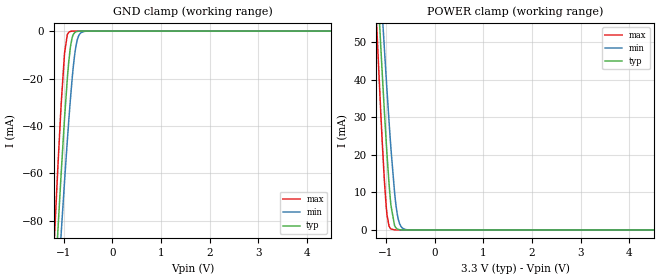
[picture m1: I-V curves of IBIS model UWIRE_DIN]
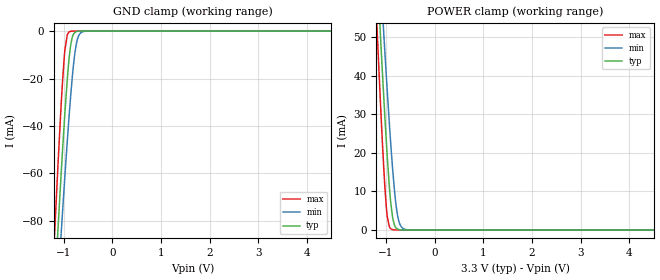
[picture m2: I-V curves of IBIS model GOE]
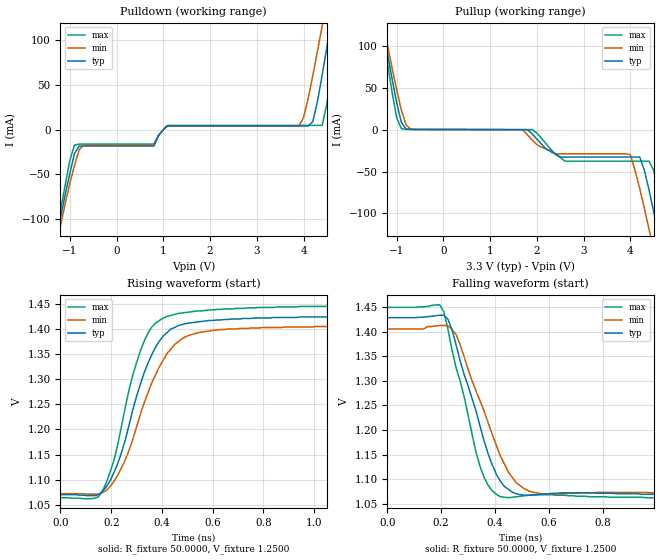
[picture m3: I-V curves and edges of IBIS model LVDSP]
| Texas Instruments Incorporated
| Precision Clock Conditioner with Integrated VCO
| Marketing part#   Voltage Range   Package-type   #pins/pkg drawing
| LMK03001   3.15V - 3.45V   LLP   48-pin SQ
[IBIS Ver]   4.1
[File name]   lmk03001.ibs
[File Rev]   1.4
[Date]   01/28/2014
[Source]   Model built from spectre simulations at:
   Texas Instruments Incorporated.
   Analog-eLab, HPA
   12500 TI Blvd
   Dallas, TX -75243
   For Support e-mail: elab_ibis@list.ti.com
[Notes]   Revision History
   Rev 1.2: 01/28/2014
   - Add uWIRE and GOE buffers, update pin assignments
   Rev 1.0: 3/26/2008
   PullUp and Pulldown non-monotonic for LVPECL and REFOUT models
   LVPECL simulation recommendation:
   It is recommended that a small (1nF or less) AC coupling cap
   be used. Larger values will result in long settling times
[Disclaimer]  This model is designed as an aid for customers of Texas Instruments
 TI and its licensors and suppliers make no warranties, either expressed
 or implied, with respect to this  model, including the warranties of
 merchantability or fitness for a particular purpose.
 The model is provided solely on an "as is" basis. The entire risk as to
 its quality and performance is with the customer.
[Copyright] (C)Copyright 2014 Texas Instruments Incorporated.
[Component]  LMK03001
[Manufacturer]  National Semiconductor Corp
[Package]
|   typ   min   max
R_pkg   0.645   0.430   0.859
L_pkg   1.735nH   1.110nH   2.360nH
C_pkg   0.0455pF   0.037pF   0.054pF
[Pin]   signal_name   model_name   R_pin   L_pin   C_pin
1   GND   GND   0.643   1.770nH   0.054pF
2   Fout   NC   0.531   1.430nH   0.041pF
3   VCC1   POWER   0.482   1.270nH   0.039pF
4   CLKuWire   UWIRE_DIN   0.445   1.160nH   0.039pF
5   DATAuWire   UWIRE_DIN   0.430   1.110nH   0.039pF
6   LEuWire   UWIRE_DIN   0.448   1.160nH   0.039pF
7   NC   NC   0.525   1.390nH   0.043pF
8   VCC2   POWER   0.520   1.370nH   0.039pF
9   LDObyp1   POWER   0.459   1.110nH   0.041pF
10   LDObyp2   POWER   0.462   1.190nH   0.039pF
11   GOE   GOE   0.464   1.220nH   0.041pF
12   LD   NC   0.512   1.390nH   0.053pF
13   VCC3   NC   0.523   1.430nH   0.051pF
14   CLKout0   LVDSP   0.507   1.360nH   0.039pF
15   CLKout0*   LVDSN   0.462   1.220nH   0.037pF
16   VCC4   POWER   0.448   1.170nH   0.037pF
17   CLKout1   LVDSP   0.434   1.120nH   0.037pF
18   CLKout1*   LVDSN   0.443   1.150nH   0.037pF
19   VCC5   POWER   0.470   1.230nH   0.037pF
20   CLKout2   LVDSP   0.505   1.330nH   0.038pF
21   CLKout2*   LVDSN   0.585   1.560nH   0.037pF
22   VCC6   POWER   0.643   1.750nH   0.038pF
23   CLKout3   LVPECLP   0.688   1.900nH   0.039pF
24   CLKout3*   LVPECLN   0.767   2.150nH   0.051pF
25   GND   GND   0.859   2.360nH   0.055pF
26   VCC7   POWER   0.802   2.150nH   0.041pF
27   SYNC*   NC   0.755   2.010nH   0.040pF
28   OSCin   OSCINP   0.725   1.930nH   0.040pF
29   OSCin*   OSCINN   0.711   1.890nH   0.040pF
30   VCC8   POWER   0.710   1.880nH   0.039pF
31   VCC9   POWER   0.745   1.900nH   0.041pF
32   Cpout   NC   0.722   1.920nH   0.040pF
33   VCC10   POWER   0.739   1.960nH   0.040pF
34   NC   NC   0.767   2.050nH   0.040pF
35   NC   NC   0.806   2.170nH   0.041pF
36   BIAS   POWER   0.847   2.330nH   0.054pF
37   VCC11   POWER   0.839   2.340nH   0.051pF
38   CLKout4   LVPECLP   0.821   2.250nH   0.040pF
39   CLKout4*   LVPECLN   0.752   2.030nH   0.038pF
40   VCC12   POWER   0.707   1.900nH   0.038pF
41   CLKout5   LVPECLP   0.670   1.780nH   0.039pF
42   CLKout5*   LVPECLN   0.623   1.650nH   0.038pF
43   VCC13   POWER   0.608   1.610nH   0.039pF
44   CLKout6   LVPECLP   0.606   1.600nH   0.039pF
45   CLKout6*   LVPECLN   0.627   1.660nH   0.038pF
46   VCC14   POWER   0.659   1.760nH   0.039pF
47   CLKout7   LVPECLP   0.695   1.880nH   0.040pF
48   CLKout7*   LVPECLN   0.753   2.080nH   0.051pF
49   DAP   NC
[Diff pin]  inv_pin  vdiff  tdelay_typ  tdelay_min  tdelay_max
14 15   0.0V   0.0s   0.0s   0.0s
17 18   0.0V   0.0s   0.0s   0.0s
20 21   0.0V   0.0s   0.0s   0.0s
23 24   0.0V   0.0s   0.0s   0.0s
28 29   200mV   0.0s   0.0s   0.0s
38 39   0.0V   0.0s   0.0s   0.0s
41 42   0.0V   0.0s   0.0s   0.0s
44 45   0.0V   0.0s   0.0s   0.0s
47 48   0.0V   0.0s   0.0s   0.0s
[Package Model] 48 LLP for LMK03001ISQ AC model at 5 GHz
[Define Package Model]  48 LLP for LMK03001ISQ AC model at 5 GHz
[Manufacturer]   National Semiconductor Corporation
[OEM]   NA
[Description]   48 LLP for LMK03001ISQ, full model
[Number Of Pins]   49
[Pin Numbers]
   1   |   1 = 1
   2   |   2 = 2
   3   |   3 = 3
   4   |   4 = 4
   5   |   5 = 5
   6   |   6 = 6
   7   |   7 = 7
   8   |   8 = 8
   9   |   9 = 9
  10   |  10 = 10
  11   |  11 = 11
  12   |  12 = 12
  13   |  13 = 13
  14   |  14 = 14
  15   |  15 = 15
  16   |  16 = 16
  17   |  17 = 17
  18   |  18 = 18
  19   |  19 = 19
  20   |  20 = 20
  21   |  21 = 21
  22   |  22 = 22
  23   |  23 = 23
  24   |  24 = 24
  25   |  25 = 25
  26   |  26 = 26
  27   |  27 = 27
  28   |  28 = 28
  29   |  29 = 29
  30   |  30 = 30
  31   |  31 = 31
  32   |  32 = 32
  33   |  33 = 33
  34   |  34 = 34
  35   |  35 = 35
  36   |  36 = 36
  37   |  37 = 37
  38   |  38 = 38
  39   |  39 = 39
  40   |  40 = 40
  41   |  41 = 41
  42   |  42 = 42
  43   |  43 = 43
  44   |  44 = 44
  45   |  45 = 45
  46   |  46 = 46
  47   |  47 = 47
  48   |  48 = 48
  49   |  49 = DAP
[Model Data]
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[End Model Data]
[End Package Model]
| Models and submodels in the file (8): UWIRE_DIN (Input), GOE (Input), LVDSP (Output), LVDSN (Output), LVPECLP (Output), LVPECLN (Output), OSCINP (Input), OSCINN (Input)
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|   Model   UWIRE_DIN
[Model] UWIRE_DIN
Model_type Input
Vinh = 0.4V
Vinl = 1.6V
C_comp   0.1674p   0.1674pF   0.1674pF
[Voltage Range]   3.3   3.15   3.45
[Temperature Range]   45   125   -40
[Power Clamp Reference]   3.3   3.15   3.45
[GND Clamp Reference]   0   0   0
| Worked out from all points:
|   GND clamp passes 1 mA (typ) near -0.79 V on its own axis
|   POWER clamp passes 1 mA (typ) near -0.82 V on its own axis
[GND Clamp]
|   Voltage   I(typ)   I(min)   I(max)
-3.3V     -965.6mA   -893.6mA   -1.069A
-1.191V   -112.1mA   -132.7mA   -88.59mA
-1.117V   -84.4mA    -107.7mA   -57.4mA
-1.048V   -59.55mA   -84.92mA   -30.5mA
-978.5mV  -36.37mA   -62.95mA   -9.221mA
-924mV    -20.4mA    -46.56mA   -1.598mA
-859.7mV  -6.75mA    -28.81mA   -125.9uA
-795.3mV  -1.278mA   -14.16mA   -6.168uA
-735.9mV  -231.4uA   -5.307mA   -322.1nA
-681.5mV  -39.54uA   -1.674mA   -19.32nA
-577.5mV  -943.2nA   -148.2uA   0A
6.595V    0A         0A         0A
[POWER Clamp]
|   Voltage   I(typ)   I(min)   I(max)
-3.3V     638.8mA    590.5mA    708.3mA
-1.196V   70.39mA    83.75mA    55.37mA
-1.107V   48.47mA    63.9mA     30.8mA
-1.077V   41.42mA    57.43mA    23.19mA
-1.038V   32.31mA    48.95mA    13.93mA
-978.5mV  19.65mA    36.67mA    3.829mA
-899.2mV  6.493mA    21.57mA    264.8uA
-825mV    1.174mA    9.968mA    10.77uA
-765.6mV  254.2uA    3.922mA    572.9nA
-701.3mV  35.15uA    1.11mA     20.98nA
-582.5mV  494.5nA    81.77uA    0A
6.595V    0A         0A         0A
|   Model GOE
[Model]   GOE
Model_type   Input
Vinl = 0.4
Vinh = 1.6
|   typ   min   max
C_comp   0.3093pF   0.3093pF   0.3093pF
[Voltage Range]   3.3   3.125   3.465
[Temperature Range]   45   125   -40
[Power Clamp Reference]   3.3   3.125   3.465
[GND Clamp Reference]   0   0   0
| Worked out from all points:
|   GND clamp passes 1 mA (typ) near -0.79 V on its own axis
|   POWER clamp passes 1 mA (typ) near -0.82 V on its own axis
[GND Clamp]
|   Voltage   I(typ)   I(min)   I(max)
-3.3V     -965.6mA   -893.6mA   -1.069A
-1.181V   -108.3mA   -129.3mA   -84.35mA
-1.112V   -82.59mA   -106mA     -55.39mA
-1.043V   -57.82mA   -83.32mA   -28.72mA
-973.5mV  -34.81mA   -61.42mA   -8.124mA
-924mV    -20.4mA    -46.56mA   -1.597mA
-884.4mV  -11.09mA   -35.36mA   -347uA
-825mV    -2.889mA   -20.4mA    -26.1uA
-745.8mV  -310.8uA   -6.404mA   -528.4nA
-676.5mV  -33.31uA   -1.499mA   -14.52nA
-577.5mV  -943.1nA   -148.2uA   0A
6.59V     0A         0A         0A
[POWER Clamp]
|   Voltage   I(typ)   I(min)   I(max)
-3.3V     638.8mA    590.5mA    708.3mA
-1.191V   69.15mA    82.63mA    53.96mA
-1.181V   66.68mA    80.4mA     51.15mA
-1.102V   47.28mA    62.82mA    29.5mA
-1.033V   31.21mA    47.91mA    12.87mA
-993.3mV  22.67mA    39.68mA    5.73mA
-933.9mV  11.5mA     27.94mA    888.7uA
-864.6mV  3.112mA    15.73mA    67.37uA
-805.2mV  711.5uA    7.563mA    4.089uA
-745.8mV  145.3uA    2.701mA    212.4nA
-577.5mV  412.5nA    72uA       0A
6.59V     0A         0A         0A
|   Model LVDSP
[Model]  LVDSP
Model_type Output
Polarity   Non-Inverting
Vmeas =  1.2780V
Rref =   50.0000
Vref =   1.2500V
C_comp   1.6000pF   1.6000pF   1.6000pF
[Temperature Range]   25.0000   85.0000   -40.0000
[Voltage Range]   3.3000V   3.1500V   3.4500V
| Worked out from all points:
|   slope of the pullup table from 0 to 0.495 V, typ, clamps not added: 9.98 kohm
|   rising waveform, R_fixture 50.0000, V_fixture 1.2500: 20-80 % time 134ps typ, 152ps min, 115ps max; typ from 1.07 V to 1.43 V
|   falling waveform, R_fixture 50.0000, V_fixture 1.2500: 20-80 % time 119ps typ, 137ps min, 101ps max; typ from 1.43 V to 1.07 V
[Pulldown]
|Voltage   I(typ)   I(min)   I(max)
-3.45V    -669.4mA   -638.7mA   -724mA
-1.3V     -126.3mA   -133.2mA   -120mA
-900mV    -26.71mA   -39.95mA   -17.23mA
-700mV    -18.3mA    -16.89mA   -16.07mA
800mV     -18.3mA    -16.89mA   -16.07mA
1.1V      4.237mA    3.877mA    4.82mA
3.9V      4.237mA    3.877mA    4.82mA
4.2V      9.056mA    60.8mA     4.82mA
4.4V      61.28mA    116.4mA    4.82mA
4.6V      124.2mA    174mA      63.07mA
4.8V      189.4mA    232.6mA    137mA
6.9V      832.6mA    800.9mA    875.6mA
[Pullup]
|Voltage   I(typ)   I(min)   I(max)
-3.45V    832.6mA    755.7mA    934.3mA
-1.3V     124.2mA    130.7mA    118.2mA
-900mV    9.056mA    23.5mA     1.096mA
-700mV    356.2uA    687.6uA    401.7uA
1.9V      -5.159mA   -12.12mA   33.99uA
2.6V      -32.65mA   -28.75mA   -37.57mA
4V        -32.65mA   -29.82mA   -37.57mA
4.2V      -32.65mA   -70.34mA   -37.57mA
4.4V      -72.21mA   -119.1mA   -37.57mA
4.6V      -125.3mA   -170.8mA   -75.8mA
4.8V      -181.4mA   -223.8mA   -134.7mA
6.9V      -666.4mA   -669.2mA   -681mA
[Ramp]
| variable   typ   min   max
dV/dt_r  0.2150/0.1345n   0.2004/0.1510n   0.2300/0.1137n
dV/dt_f  0.2172/0.1181n   0.2037/0.1385n   0.2318/0.1004n
R_load = 50.00
[Rising Waveform]
R_fixture= 50.0000
V_fixture= 1.2500
V_fixture_min= 1.2500
V_fixture_max= 1.2500
|time   V(typ)   V(min)   V(max)
0s        1.07V      1.072V     1.064V
165ps     1.076V     1.074V     1.077V
225ps     1.131V     1.108V     1.168V
270ps     1.208V     1.158V     1.278V
315ps     1.29V      1.23V      1.356V
360ps     1.349V     1.293V     1.404V
405ps     1.386V     1.338V     1.422V
480ps     1.409V     1.381V     1.432V
630ps     1.418V     1.399V     1.439V
1.485ns   1.426V     1.406V     1.448V
[Falling Waveform]
R_fixture= 50.0000
V_fixture= 1.2500
V_fixture_min= 1.2500
V_fixture_max= 1.2500
|time   V(typ)   V(min)   V(max)
0s        1.429V     1.406V     1.45V
195ps     1.434V     1.413V     1.455V
225ps     1.426V     1.413V     1.406V
255ps     1.375V     1.395V     1.328V
345ps     1.207V     1.259V     1.125V
375ps     1.151V     1.214V     1.087V
420ps     1.096V     1.147V     1.064V
480ps     1.07V      1.092V     1.064V
570ps     1.069V     1.07V      1.068V
1.485ns   1.069V     1.071V     1.06V
